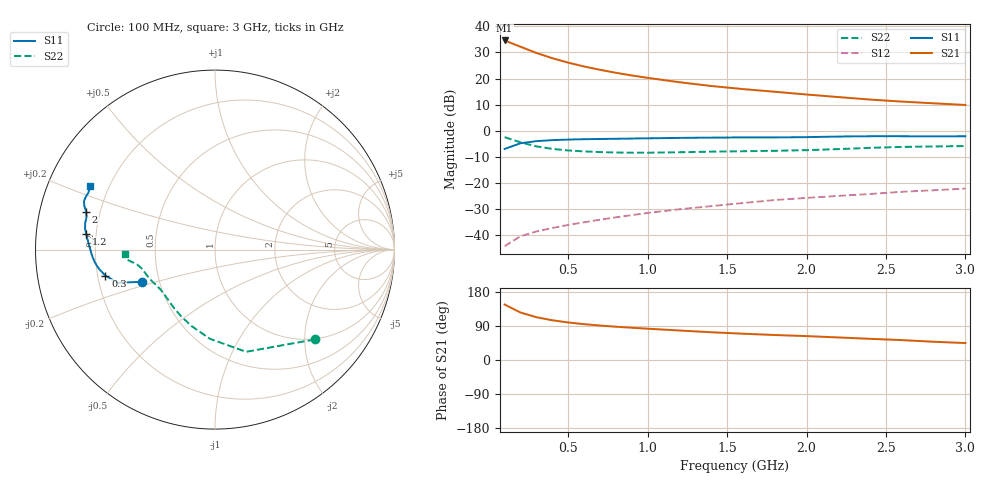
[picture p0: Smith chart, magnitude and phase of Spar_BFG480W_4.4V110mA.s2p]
! Filename: 4_4110BFG480.001
! Title: BFG480W
! Bias: Vce=4.4V; Ic=110mA
! Company: NXP Semiconductors NL
! User: Quality&Reliability T&D
! Measure time: 10 Nov 1999 / 12:07:16
#  MHz  S  MA  R 50
! Freq  S11  S21  S12  S22  :
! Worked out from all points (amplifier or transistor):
!   20 points, 100 MHz to 3 GHz, reference 50 ohm
!   highest |S21| = 34.6 dB at 100 MHz (marker M1)
!   |S21| within 3 dB of that: start of sweep to 224.5 MHz
!   unconditionally stable (mu >= 1): 687.5 MHz to end of sweep
!   at 400 MHz: K = 0.83, MSG = 32.6 dB, |S12| = -37.4 dB
!   at 1.2 GHz: K = 1.08, MAG = 22.7 dB, |S12| = -30.2 dB
!   at 3 GHz: K = 1.05, MAG = 14.7 dB, |S12| = -22.3 dB
!   S11 on the Smith chart (normalised r, x): 100 MHz: 0.40, -0.18; 300 MHz: 0.23, -0.11; 1.2 GHz: 0.16, +0.06; 2 GHz: 0.15, +0.14; 3 GHz: 0.13, +0.24
100  0.4438 -156.2  53.79 146.5  0.006032 68.8  0.7477 -42.0
200  0.5713 -161.1  40.72 125.2  0.009342 60.4  0.5952 -73.1
300  0.6275 -166.6  30.98 112.9  0.01155 59.7  0.498 -93.2
400  0.6556 -170.6  24.54 104.9  0.01345 61.5  0.4452 -107.2
500  0.672 -173.7  20.18 99.0  0.01541 63.9  0.4159 -117.3
600  0.6825 -176.3  17.02 94.6  0.01735 66.0  0.3983 -124.7
700  0.6898 -178.5  14.7 90.9  0.01944 68.0  0.3869 -130.5
800  0.6962 179.5  12.89 87.8  0.0216 69.6  0.3798 -135.4
900  0.7038 177.6  11.45 85.1  0.02378 71.5  0.3761 -139.6
1000  0.7101 175.9  10.29 82.6  0.02621 72.6  0.3761 -143.4
1200  0.7239 172.9  8.49 77.9  0.03084 74.1  0.3836 -149.4
1400  0.7337 170.7  7.186 73.2  0.0354 75.0  0.3943 -153.9
1600  0.7384 168.3  6.266 69.4  0.04065 75.7  0.4012 -157.3
1800  0.7384 165.7  5.568 66.0  0.04638 76.2  0.4092 -161.0
2000  0.7485 163.6  4.93 63.0  0.05102 76.9  0.4209 -165.4
2200  0.7685 161.4  4.4 59.5  0.05572 76.6  0.4411 -169.1
2400  0.7782 159.7  3.943 55.9  0.06059 76.1  0.4661 -171.4
2600  0.7781 158.1  3.604 52.5  0.06674 75.5  0.4861 -172.9
2800  0.7735 155.8  3.342 48.1  0.07153 74.0  0.4961 -174.6
3000  0.7783 153.1  3.103 44.7  0.07691 73.2  0.5041 -177.5
